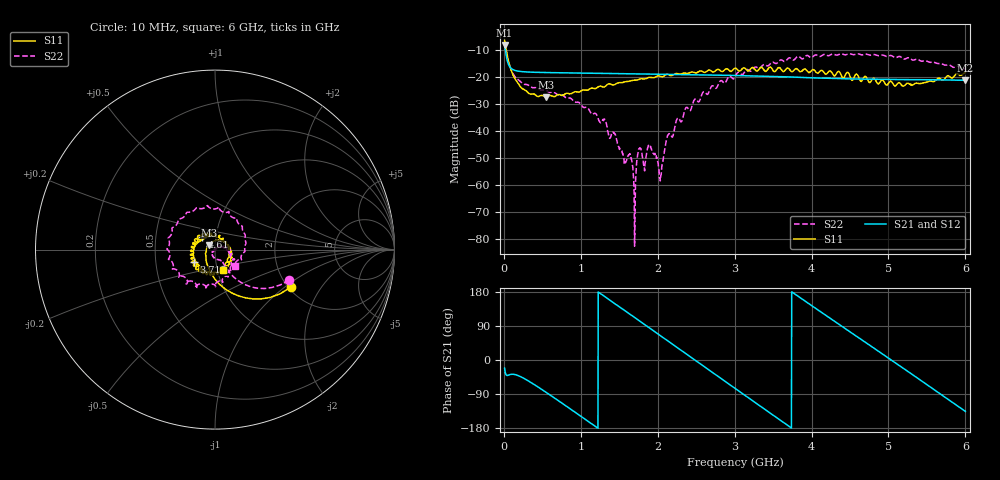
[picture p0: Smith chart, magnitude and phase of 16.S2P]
!Agilent Technologies,E5071C,MY46316741,A.11.02
!Date: Tue Oct 20 14:45:23 2020
!Data & Calibration Information:
!Freq	S11:SOLT4(ON)	S21:SOLT4(ON)	S12:SOLT4(ON)	S22:SOLT4(ON)
!PortZ  Port1:50+j0  Port2:50+j0
!Above PortZ is port z conversion or system Z0 setting when saving the data.
!When reading, reference impedance value at option line is always used.
# Hz S dB R 50
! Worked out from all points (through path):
!   1561 points, 10 MHz to 6 GHz, reference 50 ohm
!   highest |S21| = -8.15 dB at 10 MHz (marker M1); lowest = -21.3 dB at 6 GHz (marker M2)
!   group delay of S21, straight-line fit = 392 ps
!   lowest |S11| = -27.5 dB at 543.7 MHz (marker M3), VSWR 1.09, Z = 46.7 + j2.37 ohm
!   |S11| at or under -10 dB: 30.02 MHz to end of sweep
!   |S22| runs from -82.6 to -7.0 dB; largest |S21 - S12| = 0.0042
!   S11 on the Smith chart (normalised r, x): 10 MHz: 2.08, -1.11; 3.715 GHz: 0.78, -0.11; 4.61 GHz: 0.86, +0.12; 6 GHz: 1.06, -0.25
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1e7  -6.51 -26.0  -8.15 -21.8  -8.24 -21.7  -7.02 -22.5
7.14359e7  -15.34 -88.4  -15.98 -39.0  -16.01 -38.9  -15.52 -56.8
2.135064e8  -23.54 -138.6  -17.97 -43.5  -18.01 -43.5  -21.67 -58.0
5.437244e8  -27.49 143.1  -18.38 -84.5  -18.40 -84.5  -24.89 -78.7
1.012173e9  -25.05 69.7  -18.59 -150.0  -18.62 -150.2  -30.63 -118.9
1.311673e9  -23.64 36.2  -18.70 167.4  -18.72 167.2  -35.70 -143.6
1.576615e9  -21.81 11.8  -18.85 129.8  -18.88 129.6  -51.66 -156.6
1.638051e9  -21.54 5.8  -18.87 121.0  -18.89 120.9  -48.38 -122.9
1.695647e9  -21.20 1.6  -18.88 112.8  -18.91 112.7  -68.26 -18.2
1.764763e9  -20.82 -5.7  -18.91 103.0  -18.93 102.8  -46.26 -91.9
1.826199e9  -20.75 -9.7  -18.92 94.2  -18.96 94.0  -53.15 79.7
1.902994e9  -20.17 -15.8  -18.95 83.1  -18.99 82.9  -45.86 -70.1
2.006667e9  -19.57 -24.8  -19.03 68.3  -19.05 68.2  -52.27 144.1
2.045064e9  -19.88 -26.9  -19.05 62.9  -19.07 62.8  -56.14 79.6
2.129538e9  -19.02 -34.2  -19.06 50.9  -19.08 50.7  -41.64 67.8
2.367603e9  -18.65 -53.3  -19.17 16.9  -19.20 16.6  -31.38 44.7
3.005e9  -16.80 -100.9  -19.46 -74.7  -19.51 -74.9  -20.08 -27.8
3.715353e9  -17.27 -148.6  -19.99 -176.2  -20.04 -176.3  -12.93 -102.4
4.007173e9  -17.41 -178.4  -20.34 142.7  -20.36 142.6  -12.77 -139.2
4.610013e9  -19.93 135.2  -20.78 59.1  -20.81 58.9  -11.47 152.7
5.001667e9  -22.28 71.5  -20.90 4.6  -20.92 4.5  -12.26 101.8
6e9  -18.31 -69.9  -21.25 -135.5  -21.27 -135.5  -16.71 -38.6
